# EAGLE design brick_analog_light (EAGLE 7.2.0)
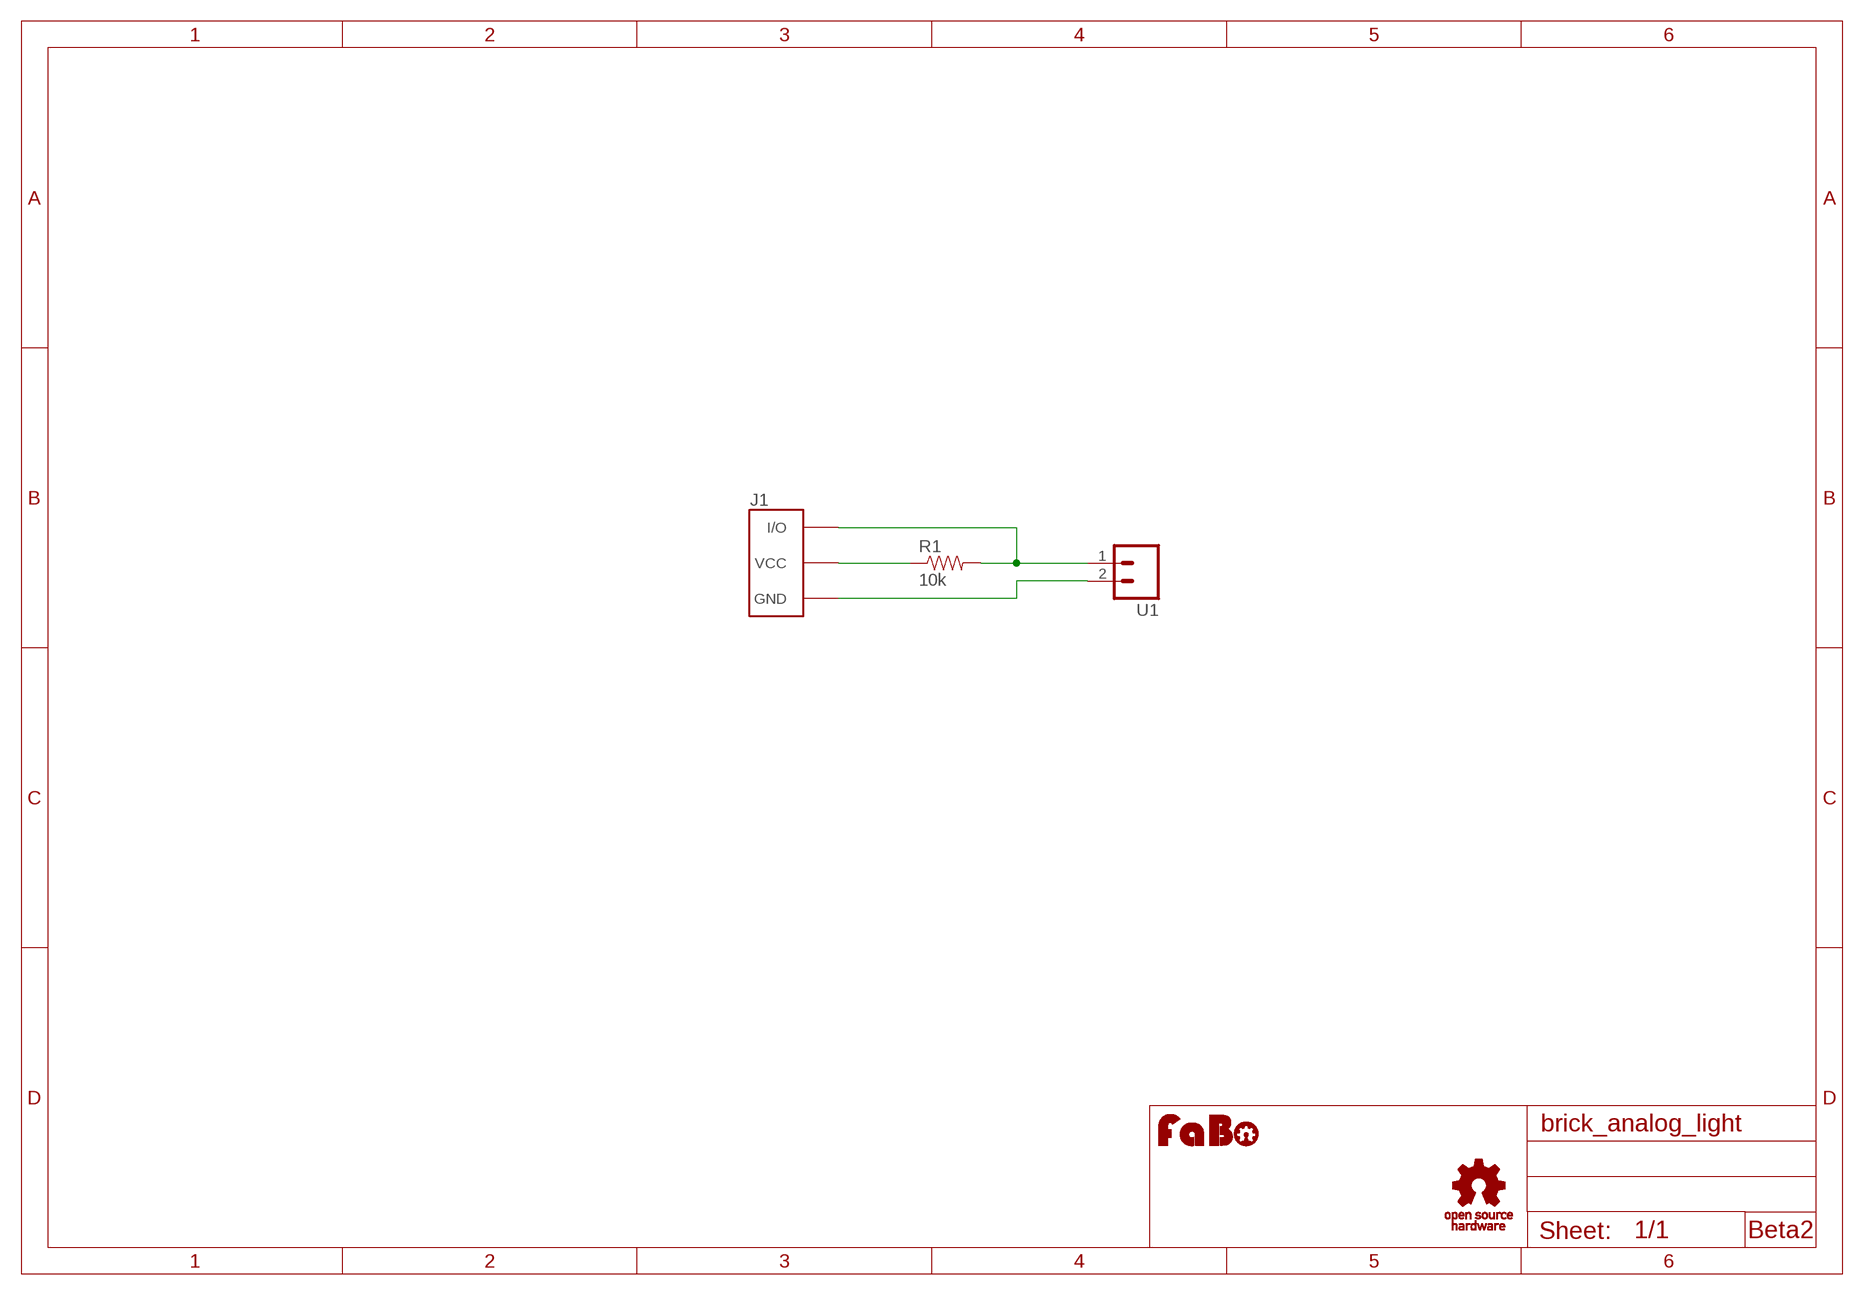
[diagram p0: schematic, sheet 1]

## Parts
J1  BRICK_3PIN  [BRICK_3PIN]
R1  10k  RES-PTH-REGULAR  [RES-AXL-REGULAR]
U1  M02NG  [1X02]
U$2  LOGO_FABO-M  [LOGO_FABO_M]
U$4  LOGO_OSHW_T-M  [LOGO_OSHW_T_M]

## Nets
GND: J1.GND U1.2
N$1: J1.VCC R1.P$1
N$2: J1.IN/OUT(I/O) R1.P$2 U1.1

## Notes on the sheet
- Beta2

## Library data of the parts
J1 = Gclue:BRICK_3PIN: FaBo Brick 3pin
R1 = Gclue:RES
U1 = SparkFun:M02NG
U$2 = FaBo:LOGO_FABO
U$4 = Gclue:LOGO_OSHW_T

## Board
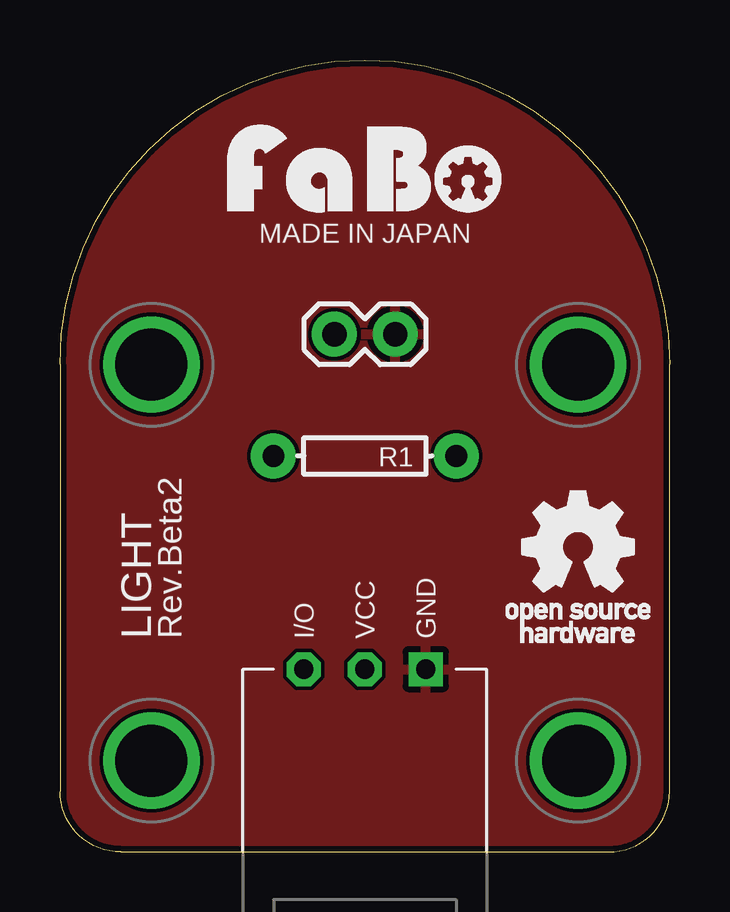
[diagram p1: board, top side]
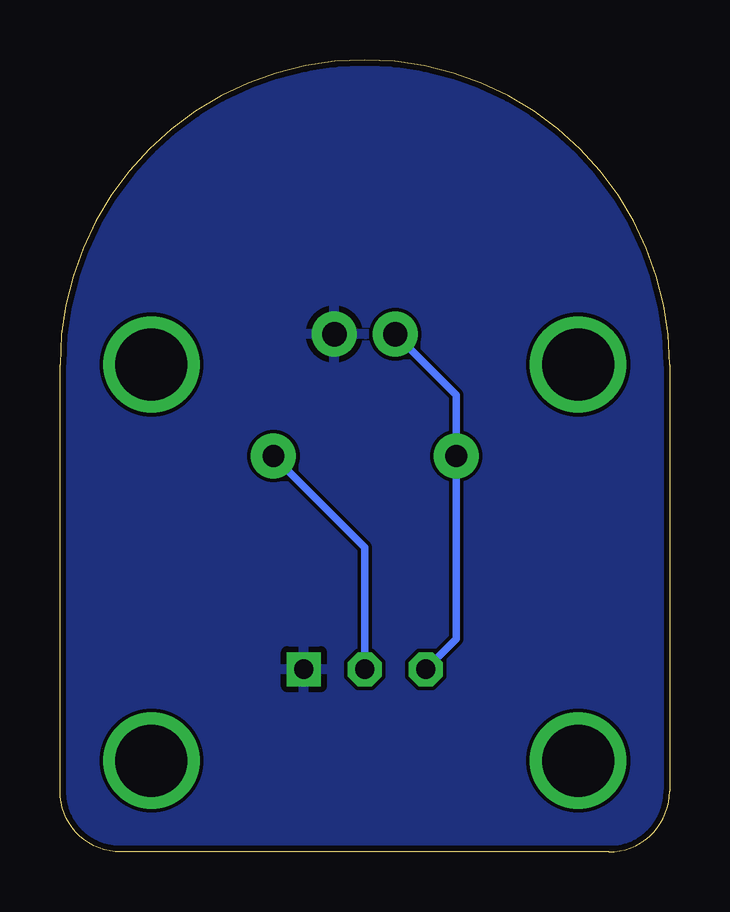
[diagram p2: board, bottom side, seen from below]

Size 25.4 x 33.02 mm. Coordinates in mm from the lower left corner, seen from the top.
Copper layers (1*16): Top 0.035mm / dielectric 1.5mm / Bottom 0.035mm
Design rules "Elecrow_2-layer_eagle_rule": minimum track width 6mil, minimum drill 12mil, track to track 6mil, track to pad 6mil, pad to pad 6mil, via to via 6mil, smd to smd 0mil, copper to edge 10mil, drill to drill 10mil, minimum pad ring 10mil, minimum via ring 6mil, stop-mask expansion 2mil, vias tented up to drill 100mil, thermal gap 10mil

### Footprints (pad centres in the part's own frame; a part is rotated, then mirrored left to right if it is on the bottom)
BRICK_3PIN = drill 0.8 pad 1.422 square: GND 2.54,-8.89 | drill 0.8 pad 1.422 octagon: IN/OUT -2.54,-8.89; VCC 0,-8.89 | drill 3 pad 3.81: P$5 -8.89,3.81; P$6 8.89,3.81; P$7 -8.89,-12.7; P$8 8.89,-12.7
RES-AXL-REGULAR = drill 0.9 pad 1.88: P$1 -3.81,0; P$2 3.81,0
1X02 = drill 1.016 pad 1.88: 1 0,0; 2 2.54,0

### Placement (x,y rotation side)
J1  12.7,16.51 0 top
R1  12.7,16.51 180 top
U1  11.43,21.59 0 top
U$2  12.7,26.67 0 top
U$4  21.59,12.7 0 top

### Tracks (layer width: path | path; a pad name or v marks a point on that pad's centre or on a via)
GND
  pour Bottom: -1.27,-1.27 26.67,-1.27 26.67,34.29 -1.27,34.29
  pour Top: -1.27,-1.27 26.67,-1.27 26.67,34.29 -1.27,34.29
N$1
  Bottom 0.305: J1.VCC 12.7,12.7 R1.P$1
N$2
  Bottom 0.305: J1.IN/OUT 8.89,8.89 R1.P$2 8.89,19.05 U1.1

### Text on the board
tPlace: MADE IN JAPAN | LIGHT | Rev.Beta2

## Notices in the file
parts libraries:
SparkFun: Licensing: CC v3.0 Share-Alike You are welcome to use this library for commercial purposes.
